FUNCTION F_CALC_LIN_CHKSUM : BYTE
VAR_INPUT
   pData:POINTER TO ARRAY[0..10] OF BYTE; // Pointer to source datafield
   nLen:BYTE;  // Number of bytes used for calculating the checksum
END_VAR
VAR
   i: BYTE; // Counter variable 
   wResult:WORD; // Resulting output value
END_VAR

wResult := BYTE_TO_WORD(pData^[0]);
FOR i := 1 TO (nLen-1) DO
   wResult := wResult + BYTE_TO_WORD(pData^[i]);
   IF wResult > 255 THEN
      wResult := wResult - 255;
   END_IF
END_FOR
F_CALC_LIN_CHKSUM := WORD_TO_BYTE(NOT(wResult));

END_FUNCTION
